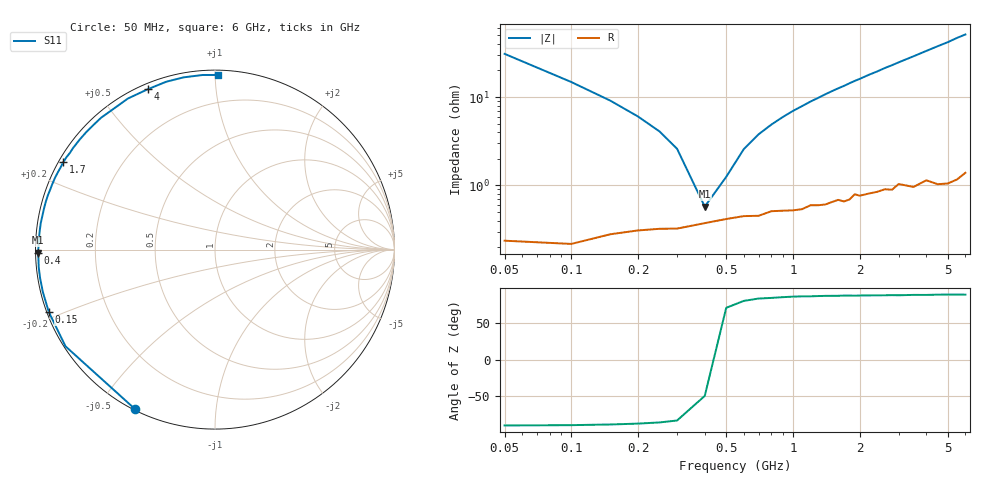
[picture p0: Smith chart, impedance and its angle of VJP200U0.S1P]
! Infineon Technologies  Discrete & RF Semiconductors
! BB 914
! Si Tuning Diode in SOT23
! VR = 0.2 V
! S-Parameters:  July  1999
# GHz  S  MA  R  50
!  f  S11
! GHz  MAG  ANG
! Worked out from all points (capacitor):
!   34 points, 50 MHz to 6 GHz, reference 50 ohm
!   read as one part to ground: C = 102 pF near 50 MHz
!   lowest |Z| = 575 mohm at 400 MHz (marker M1)
!   series resonance near 427 MHz, so ESL is about 1.4 nH
!   S11 on the Smith chart (normalised r, x): 50 MHz: 0.00, -0.62; 150 MHz: 0.01, -0.18; 400 MHz: 0.01, -0.01; 1.7 GHz: 0.01, +0.27; 4 GHz: 0.02, +0.66; 6 GHz: 0.03, +1.02
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0.05  0.9931 -116.8
0.1  0.992 -147.1
0.15  0.9892 -159.4
0.2  0.9879 -166.3
0.25  0.9872 -170.7
0.3  0.9871 -174.1
0.4  0.9851 -179.0
0.5  0.9835 177.3
0.6  0.9822 174.2
0.7  0.9821 171.4
0.8  0.98 168.9
1  0.9797 164.2
1.2  0.9771 159.9
1.4  0.977 155.8
1.6  0.9745 151.9
1.7  0.9757 150.1
1.8  0.9747 148.1
2.2  0.9717 140.8
2.4  0.971 137.5
2.6  0.9698 133.9
2.8  0.9709 130.8
3  0.9672 127.5
3.5  0.9716 120.0
4  0.9688 112.8
4.5  0.9739 106.2
5  0.9755 100.3
5.5  0.9753 94.0
6  0.9731 88.9
